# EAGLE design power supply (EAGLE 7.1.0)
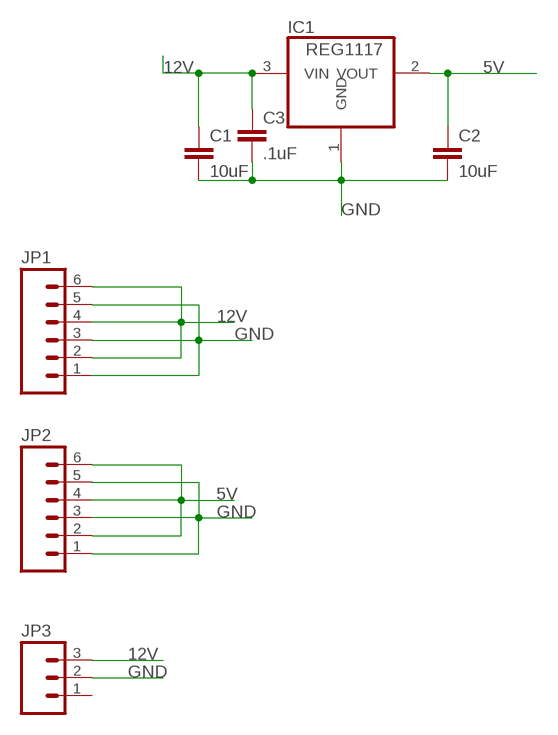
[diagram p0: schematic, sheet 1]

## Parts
C1  10uF  CAP1206  [1206]
C2  10uF  CAP1206  [1206]
C3  .1uF  CAP1206  [1206]
IC1  REG1117  [SOT223]
JP1  M06LONGPADS  [1X06_LONGPADS]
JP2  M06LONGPADS  [1X06_LONGPADS]
JP3  M03LOCK_LONGPADS  [1X03_LOCK_LONGPADS]

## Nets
5V: C2.1 IC1.2(VOUT) JP2.2 JP2.4 JP2.6
12V: C1.1 C3.1 IC1.3(VIN) JP1.2 JP1.4 JP1.6 JP3.3
GND: C1.2 C2.2 C3.2 IC1.1(GND) JP1.1 JP1.3 JP1.5 JP2.1 JP2.3 JP2.5 JP3.2
Unconnected: JP3.1

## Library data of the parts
C1-C3 = 01_SparkFun:CAP: Capacitor
IC1 = burr-brown:REG1117: 800mA and 1A Low Dropout (LDO) Positive Regulator 1.8V, 2.5V, 2.85V, 3.3V, 5V, and Adj; MPN: REG1117; OC_FARNELL: 1097566; OC_NEWARK: 14P6981
JP1 JP2 = 01_SparkFun:M06: Header 6 Standard 6-pin 0.1" header. Use with straight break away headers (SKU : PRT-00116), right angle break away headers (PRT-00553), swiss pins (PRT-00743), machine pins (PRT-00117), and female headers (PRT-00115). Molex polarized connector foot print use with SKU : PRT-08094 with associated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
JP3 = 01_SparkFun:M03: Header 3 Standard 3-pin 0.1" header. Use with straight break away headers (SKU : PRT-00116), right angle break away headers (PRT-00553), swiss pins (PRT-00743), machine pins (PRT-00117), and female headers (PRT-00115). Molex polarized connector foot print use with SKU : PRT-08232 with associated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

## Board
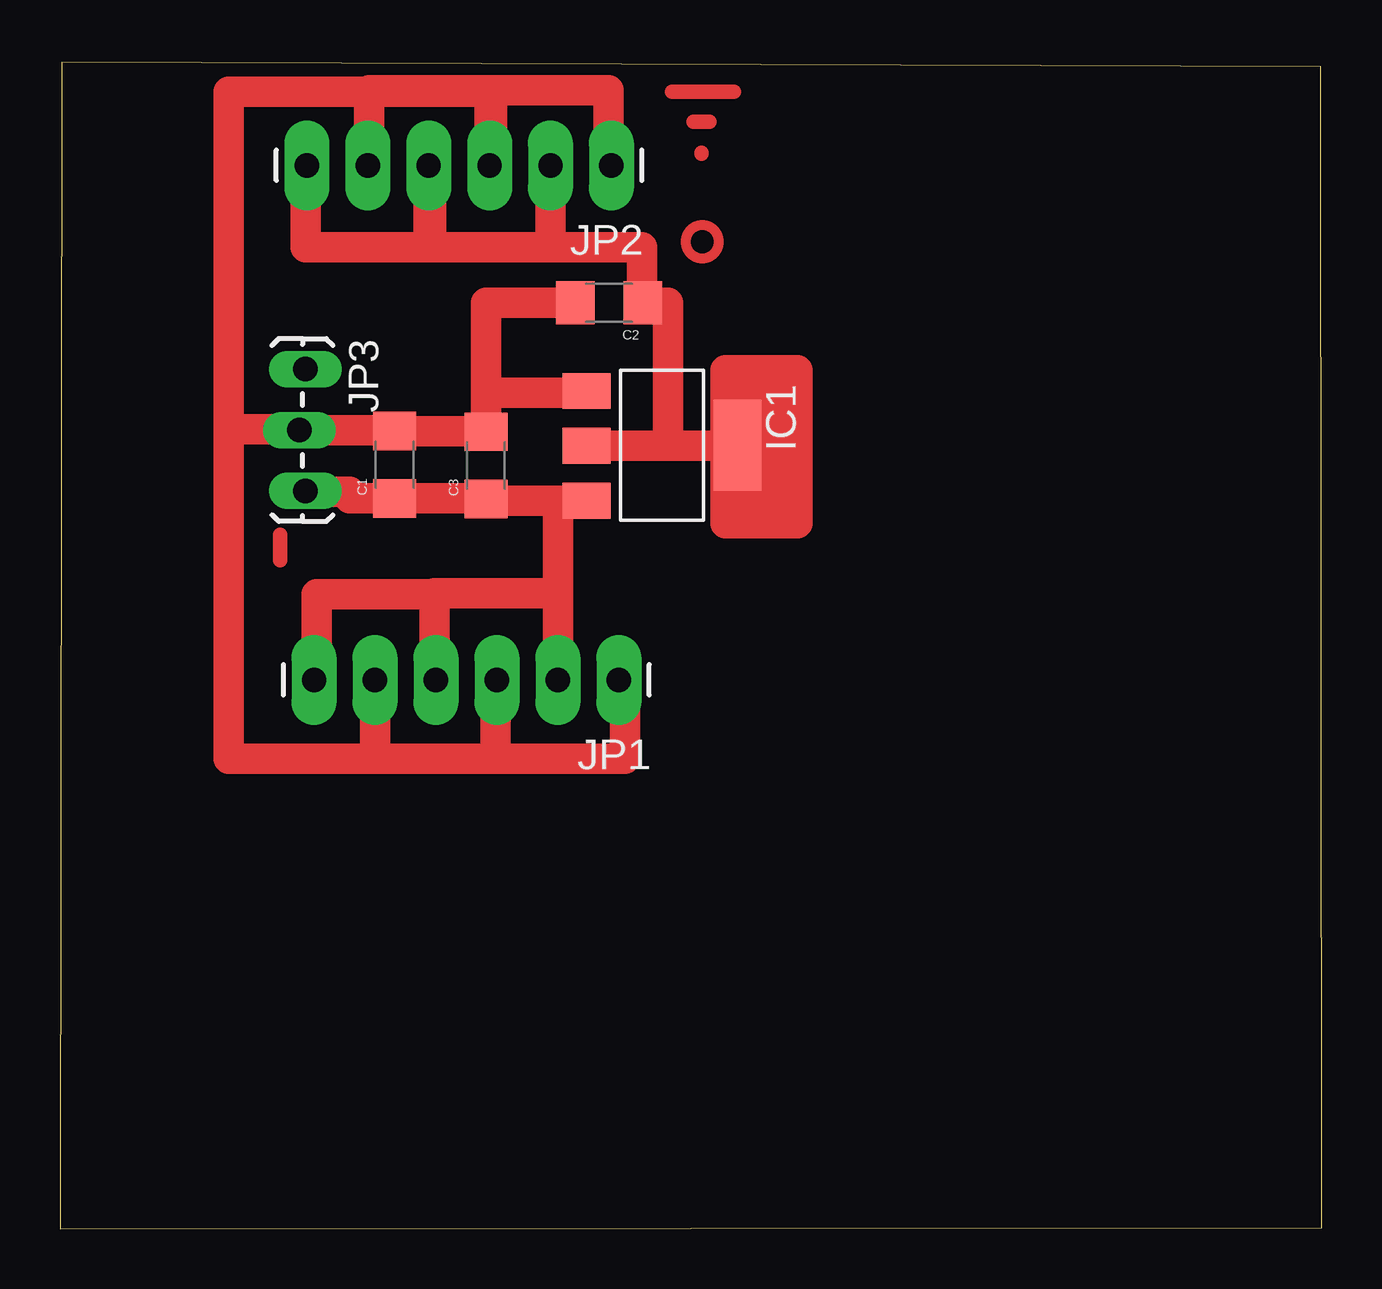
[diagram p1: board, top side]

Size 52.6 x 48.61 mm. Coordinates in mm from the lower left corner, seen from the top.
Outline: 0,0 52.6,0.03 52.55,48.4 0.08,48.61 0,0
Copper layers (1*16): Top 0.035mm / dielectric 1.5mm / Bottom 0.035mm
Design rules "default *": minimum track width 14mil, minimum drill 24mil, track to track 15mil, track to pad 15mil, pad to pad 15mil, via to via 15mil, smd to smd 15mil, copper to edge 40mil, drill to drill 8mil, minimum pad ring 10mil, minimum via ring 8mil, stop-mask expansion 4mil, vias tented up to drill 0mil, thermal gap 10mil

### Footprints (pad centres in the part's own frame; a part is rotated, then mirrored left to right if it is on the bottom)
1206 = smd 1.6 x 1.8: 1 -1.4,0; 2 1.4,0
SOT223 = smd 1.499 x 2.007: 1 -2.261,-3.15; 2 0.025,-3.15; 3 2.311,-3.15 | smd 3.81 x 2.007: 4 0,3.15
1X06_LONGPADS = drill 1.016 pad 1.88 long: 1 0,0; 2 2.54,0; 3 5.08,0; 4 7.62,0; 5 10.16,0; 6 12.7,0
1X03_LOCK_LONGPADS = drill 1.016 long: 1 0,0; 2 2.54,-0.254; 3 5.08,0

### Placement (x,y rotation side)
C1  13.94,31.83 90 top
C2  22.89,38.58 180 top
C3  17.75,31.8 90 top
IC1  25.1,32.64 270 top
JP1  23.29,22.86 180 top
JP2  22.99,44.3 180 top
JP3  10.24,35.81 270 top

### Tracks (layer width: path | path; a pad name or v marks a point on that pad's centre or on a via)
5V
  Top 1.27: IC1.2 25.35,32.61 | 25.35,32.61 27.74,32.61 | 27.74,32.61 27.74,32.59 | 27.74,32.59 27.74,29.39 30.73,29.39 30.73,35.76 27.74,35.76 27.74,32.61 | 27.74,32.59 29.67,32.59 29.67,30.38 28.68,30.38 28.68,34.82 29.74,34.82 29.74,33.38 | 25.35,32.61 25.35,38.58 C2.1 24.26,38.58 24.26,40.89 20.45,40.89 | 20.45,40.89 JP2.2 | JP2.6 10.24,44.3 10.24,40.89 15.37,40.89 JP2.4 15.47,44.3 15.47,40.89 20.45,40.89
12V
  Top 1.27: JP3.3 10.24,30.71 12.06,30.71 12.06,30.43 C1.1 17.75,30.43 C3.1 17.75,30.33 IC1.3 20.75,30.33 20.75,26.47 | 20.75,26.47 JP1.2 | JP1.4 15.62,22.86 15.62,26.44 | 20.75,26.47 15.62,26.47 15.62,26.44 | JP1.6 10.69,22.86 10.69,26.44 15.62,26.44
GND
  Top 1.27: C3.2 17.75,33.23 C1.2 13.94,33.27 JP3.2 9.98,33.3 7.04,33.3 | C3.2 17.75,34.82 21.95,34.82 IC1.1 | C2.2 17.75,38.58 C3.2 | JP2.1 22.86,44.3 22.86,47.42 17.91,47.42 | 17.91,47.42 JP2.3 18.01,44.3 18.01,47.37 7.04,47.37 7.04,33.3 | JP2.5 12.88,44.3 12.88,47.42 17.91,47.42 | JP1.5 13.13,19.58 | 13.13,19.58 7.04,19.58 7.04,33.3 | JP1.3 18.16,22.86 18.16,19.58 | 18.16,19.58 13.13,19.58 | JP1.1 23.55,22.86 23.55,19.58 18.16,19.58
N$1
  Top 0.61: 9.17,28.9 9.17,27.84
N$2
  Top 0.61: 25.5,47.37 28.09,47.37
N$3
  Top 0.61: 26.42,46.13 27.08,46.13
N$4
  Top 0.61: 26.75,44.78 26.75,44.83
(copper drawn outside any net)
  shapes: Top circle x1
